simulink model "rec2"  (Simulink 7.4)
settings: Solver=ode15s  StartTime=0.0  StopTime=0.05  MaxStep=1e-4  RelTol=1e-5  AbsTol=1e-5

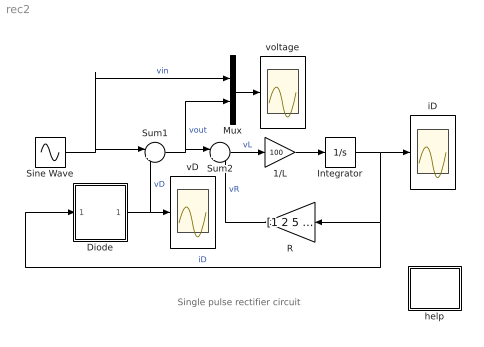
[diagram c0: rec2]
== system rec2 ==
  note: Single pulse rectifier circuit
  1/L : Gain  Gain=100  ParameterDataType=sfix(16)  ParameterScaling=2^0  OutDataType=sfix(16)  OutScaling=2^0
  Diode : Subsystem
  Integrator : Integrator
  Mux : Mux  Inputs=2
  R : Gain  Gain=[1 2 5 10]  ParameterDataType=sfix(16)  ParameterScaling=2^0  OutDataType=sfix(16)  OutScaling=2^0
  Sine Wave : Sin  Amplitude=120*sqrt(2)  Bias=0  Frequency=2*pi*60  Phase=0  Samples=10  SampleTime=0
  Sum1 : Sum  Inputs=|+-  OutDataType=sfix(16)  OutScaling=2^0
  Sum2 : Sum  Inputs=|+-  OutDataType=sfix(16)  OutScaling=2^0
  help : Subsystem
  iD : Scope
  vD : Scope
  voltage : Scope
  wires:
  1/L/1 -> Integrator/1
  Sum2/1 -> 1/L/1  "vL"
  R/1 -> Sum2/2  "vR"
  Integrator/1 -> iD/1, R/1, Diode/1(iD)  "iD"
  Sum1/1 -> Sum2/1, Mux/2  "vout"
  Sine Wave/1 -> Sum1/1, Mux/1  "vin"
  Diode/1(vD) -> Sum1/2, vD/1  "vD"
  Mux/1 -> voltage/1

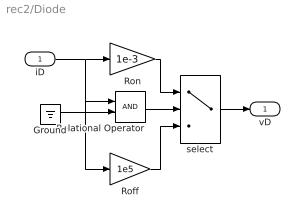
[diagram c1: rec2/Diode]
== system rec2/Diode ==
  iD : Inport  OutDataType=sfix(16)  OutScaling=2^0
  Ground : Ground
  Relational Operator : RelationalOperator
  Roff : Gain  Gain=1e5  ParameterDataType=sfix(16)  ParameterScaling=2^0  OutDataType=sfix(16)  OutScaling=2^0
  Ron : Gain  Gain=1e-3  ParameterDataType=sfix(16)  ParameterScaling=2^0  OutDataType=sfix(16)  OutScaling=2^0
  select : Switch  Threshold=0.5
  vD : Outport
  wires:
  Ground/1 -> Relational Operator/2
  Relational Operator/1 -> select/2
  Ron/1 -> select/1
  Roff/1 -> select/3
  select/1 -> vD/1
  iD/1 -> Ron/1, Relational Operator/1, Roff/1

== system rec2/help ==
